| This Model is valid for Automotive grade 3 grade Temperature Range -40C<=Tc<=95C
| Valid for DDR3/DDR3L-1866/2133 operation
| Part Number   VDDQ   Package   Architecture
| SCB13H2G160GF   1.35 +0.1/-0.067   BGA   2G bit x 16
| SCB15H2G160GF   1.5  +0.075/-0.075   BGA   2G bit x 16
[IBIS ver] 5.0
[File name]  ussxh2g16ga3.ibs
[File Rev]  1.0
[Date]   April 23, 2024
[Source] Simulation of a silicon level SPICE model
[Notes]  IBIS Characteristics for I/O Buffer
  IBIS Model Revision History: Rev 1.0:
  2024-04-23 - IBIS model file initial creation
[Disclaimer]  The IBIS models are for modeling purpose only and are subject to change without any notice. UniIC is not
  responsible for any problems the models may cause.
[Copyright] Copyright 2024 UniIC Semiconductors Corp. All rights reserved
|   Component SCB13H2G160GF
[Component] SCB13H2G160GF
[Manufacturer] UniIC Semiconductors Corp.
[Package]
| variable   typ   min   max
R_pkg   0.767   0.689   0.873
L_pkg   2.690nH   2.450nH   3.190nH
C_pkg   0.644pF   0.547pF   0.754pF
[Pin]  signal_name   model_name   R_pin   L_pin   C_pin
A1   VDDQ   Power
A2   DQU5   DQ   0.873   3.190nH   0.754pF
A3   DQU7   DQ   0.808   2.940nH   0.688pF
A7   DQU4   DQ   0.783   2.690nH   0.710pF
A8   VDDQ   Power
A9   VSS   Gnd
B1   VSS   Gnd
B2   VDD   Power
B3   VSS   Gnd
B7   DQSU#   DQ   0.767   2.730nH   0.704pF
B8   DQU6   DQ   0.826   2.890nH   0.738pF
B9   VSS   Gnd
C1   VDDQ   Power
C2   DQU3   DQ   0.800   2.760nH   0.697pF
C3   DQU1   DQ   0.759   2.780nH   0.662pF
C7   DQSU   DQ   0.729   2.680nH   0.650pF
C8   DQU2   DQ   0.739   2.750nH   0.657pF
C9   VDDQ   Power
D1   VSS   Gnd
D2   VDDQ   Power
D3   DMU   DQ   0.730   2.620nH   0.614pF
D7   DQU0   DQ   0.719   2.540nH   0.621pF
D8   VSS   Gnd
D9   VDD   Power
E1   VSS   Gnd
E2   VSS   Gnd
E3   DQL0   DQ   0.777   2.840nH   0.606pF
E7   DML   DQ   0.723   2.480nH   0.608pF
E8   VSS   Gnd
E9   VDDQ   Power
F1   VDDQ   Power
F2   DQL2   DQ   0.738   2.720nH   0.592pF
F3   DQSL   DQ   0.710   2.520nH   0.547pF
F7   DQL1   DQ   0.776   2.590nH   0.556pF
F8   DQL3   DQ   0.793   2.700nH   0.670pF
F9   VSS   Gnd
G1   VSS   Gnd
G2   DQL6   DQ   0.791   2.690nH   0.671pF
G3   DQSL#   DQ   0.689   2.450nH   0.550pF
G7   VDD   Power
G8   VSS   Gnd
G9   VSS   Gnd
H1   VREFDQ   Power
H2   VDDQ   Power
H3   DQL4   DQ   0.740   2.670nH   0.593pF
H7   DQL7   DQ   0.767   2.510nH   0.637pF
H8   DQL5   DQ   0.771   2.560nH   0.629pF
H9   VDDQ   Power
J1   NC1   NC
J2   VSS   Gnd
J3   RAS#   CA   0.738   2.460nH   0.669pF
J7   CK   CLK   0.416   1.450nH   0.409pF
J8   VSS   Gnd
J9   NC2   NC
K1   ODT   RCV_ODT   0.658   2.580nH   0.566pF
K2   VDD   Power
K3   CAS#   CA   0.762   2.490nH   0.692pF
K7   CK#   CLK   0.400   1.490nH   0.364pF
K8   VDD   Power
K9   CKE   CA   0.646   2.440nH   0.567pF
L1   NC3   NC
L2   CS#   CA   0.740   2.760nH   0.578pF
L3   WE#   CA   0.708   2.610nH   0.518pF
L7   A10_AP   CA   0.694   2.670nH   0.504pF
L8   ZQ   Power
L9   NC4   NC
M1   VSS   Gnd
M2   BA0   CA   0.762   3.000nH   0.609pF
M3   BA2   CA   0.725   2.790nH   0.545pF
M7   NC5   NC
M8   VREFCA   Power
M9   VSS   Gnd
N1   VDD   Power
N2   A3   CA   0.697   2.800nH   0.595pF
N3   A0   CA   0.654   2.720nH   0.550pF
N7   A12_BC   CA   0.691   2.550nH   0.585pF
N8   BA1   CA   0.734   3.070nH   0.562pF
N9   VDD   Power
P1   VSS   Gnd
P2   A5   CA   0.723   2.950nH   0.631pF
P3   A2   CA   0.725   2.990nH   0.598pF
P7   A1   CA   0.641   2.670nH   0.572pF
P8   A4   CA   0.721   2.780nH   0.646pF
P9   VSS   Gnd
R1   VDD   Power
R2   A7   CA   0.801   3.060nH   0.699pF
R3   A9   CA   0.712   2.920nH   0.627pF
R7   A11   CA   0.677   2.830nH   0.602pF
R8   A6   CA   0.793   3.120nH   0.708pF
R9   VDD   Power
T1   VSS   Gnd
T2   RESET#   RST_N
T3   A13   CA   0.807   2.990nH   0.695pF
T7   NC6   NC
T8   A8   CA   0.867   3.280nH   0.754pF
T9   VSS   Gnd
|IN   dq_in   dummy
|EN   dq_en   dummy
[Diff pin]  inv_pin  vdiff   tdelay_typ   tdelay_min   tdelay_max
C7   B7   0.270V   NA   NA   NA
F3   G3   0.270V   NA   NA   NA
J7   K7   0.270V   NA   NA   NA
|   Component SCB15H2G160GF
[Component] SCB15H2G160GF
[Manufacturer] UniIC Semiconductors Corp.
[Package]
| variable   typ   min   max
R_pkg   0.767   0.689   0.873
L_pkg   2.690nH   2.450nH   3.190nH
C_pkg   0.644pF   0.547pF   0.754pF
[Pin]  signal_name   model_name   R_pin   L_pin   C_pin
A1   VDDQ   Power
A2   DQU5   DQ   0.873   3.190nH   0.754pF
A3   DQU7   DQ   0.808   2.940nH   0.688pF
A7   DQU4   DQ   0.783   2.690nH   0.710pF
A8   VDDQ   Power
A9   VSS   Gnd
B1   VSS   Gnd
B2   VDD   Power
B3   VSS   Gnd
B7   DQSU#   DQ   0.767   2.730nH   0.704pF
B8   DQU6   DQ   0.826   2.890nH   0.738pF
B9   VSS   Gnd
C1   VDDQ   Power
C2   DQU3   DQ   0.800   2.760nH   0.697pF
C3   DQU1   DQ   0.759   2.780nH   0.662pF
C7   DQSU   DQ   0.729   2.680nH   0.650pF
C8   DQU2   DQ   0.739   2.750nH   0.657pF
C9   VDDQ   Power
D1   VSS   Gnd
D2   VDDQ   Power
D3   DMU   DQ   0.730   2.620nH   0.614pF
D7   DQU0   DQ   0.719   2.540nH   0.621pF
D8   VSS   Gnd
D9   VDD   Power
E1   VSS   Gnd
E2   VSS   Gnd
E3   DQL0   DQ   0.777   2.840nH   0.606pF
E7   DML   DQ   0.723   2.480nH   0.608pF
E8   VSS   Gnd
E9   VDDQ   Power
F1   VDDQ   Power
F2   DQL2   DQ   0.738   2.720nH   0.592pF
F3   DQSL   DQ   0.710   2.520nH   0.547pF
F7   DQL1   DQ   0.776   2.590nH   0.556pF
F8   DQL3   DQ   0.793   2.700nH   0.670pF
F9   VSS   Gnd
G1   VSS   Gnd
G2   DQL6   DQ   0.791   2.690nH   0.671pF
G3   DQSL#   DQ   0.689   2.450nH   0.550pF
G7   VDD   Power
G8   VSS   Gnd
G9   VSS   Gnd
H1   VREFDQ   Power
H2   VDDQ   Power
H3   DQL4   DQ   0.740   2.670nH   0.593pF
H7   DQL7   DQ   0.767   2.510nH   0.637pF
H8   DQL5   DQ   0.771   2.560nH   0.629pF
H9   VDDQ   Power
J1   NC1   NC
J2   VSS   Gnd
J3   RAS#   CA   0.738   2.460nH   0.669pF
J7   CK   CLK   0.416   1.450nH   0.409pF
J8   VSS   Gnd
J9   NC2   NC
K1   ODT   RCV_ODT   0.658   2.580nH   0.566pF
K2   VDD   Power
K3   CAS#   CA   0.762   2.490nH   0.692pF
K7   CK#   CLK   0.400   1.490nH   0.364pF
K8   VDD   Power
K9   CKE   CA   0.646   2.440nH   0.567pF
L1   NC3   NC
L2   CS#   CA   0.740   2.760nH   0.578pF
L3   WE#   CA   0.708   2.610nH   0.518pF
L7   A10_AP   CA   0.694   2.670nH   0.504pF
L8   ZQ   Power
L9   NC4   NC
M1   VSS   Gnd
M2   BA0   CA   0.762   3.000nH   0.609pF
M3   BA2   CA   0.725   2.790nH   0.545pF
M7   NC5   NC
M8   VREFCA   Power
M9   VSS   Gnd
N1   VDD   Power
N2   A3   CA   0.697   2.800nH   0.595pF
N3   A0   CA   0.654   2.720nH   0.550pF
N7   A12_BC   CA   0.691   2.550nH   0.585pF
N8   BA1   CA   0.734   3.070nH   0.562pF
N9   VDD   Power
P1   VSS   Gnd
P2   A5   CA   0.723   2.950nH   0.631pF
P3   A2   CA   0.725   2.990nH   0.598pF
P7   A1   CA   0.641   2.670nH   0.572pF
P8   A4   CA   0.721   2.780nH   0.646pF
P9   VSS   Gnd
R1   VDD   Power
R2   A7   CA   0.801   3.060nH   0.699pF
R3   A9   CA   0.712   2.920nH   0.627pF
R7   A11   CA   0.677   2.830nH   0.602pF
R8   A6   CA   0.793   3.120nH   0.708pF
R9   VDD   Power
T1   VSS   Gnd
T2   RESET#   RST_N
T3   A13   CA   0.807   2.990nH   0.695pF
T7   NC6   NC
T8   A8   CA   0.867   3.280nH   0.754pF
T9   VSS   Gnd
[Diff pin]  inv_pin  vdiff   tdelay_typ   tdelay_min   tdelay_max
C7   B7   0.270V   NA   NA   NA
F3   G3   0.270V   NA   NA   NA
J7   K7   0.270V   NA   NA   NA
[Model Selector] DQ
DQ_RON60_DDR3  DQ/ DQS RON=60ohms, for DDR3
DQ_RON60_DDR3L  DQ/ DQS RON=60ohms, for DDR3L
DQ_RON48_DDR3  DQ/ DQS RON=48ohms, for DDR3
DQ_RON48_DDR3L  DQ/ DQS RON=48ohms, for DDR3L
DQ_RON40_DDR3  DQ/ DQS RON=40ohms, for DDR3
DQ_RON40_DDR3L  DQ/ DQS RON=40ohms, for DDR3L
DQ_RON34_DDR3  DQ/ DQS RON=34ohms, for DDR3
DQ_RON34_DDR3L  DQ/ DQS RON=34ohms, for DDR3L
DQ_RCV_ODTOFF_DDR3  DQ/DM RCV ODTOFF, for DDR3
DQ_RCV_ODTOFF_DDR3L  DQ/DM RCV ODTOFF, for DDR3L
DQ_RCV_ODT120_DDR3  DQ/DM RCV ODT120, for DDR3
DQ_RCV_ODT120_DDR3L  DQ/DM RCV ODT120, for DDR3L
DQ_RCV_ODT60_DDR3  DQ/DM RCV ODT60, for DDR3
DQ_RCV_ODT60_DDR3L  DQ/DM RCV ODT60, for DDR3L
DQ_RCV_ODT40_DDR3  DQ/DM RCV ODT40, for DDR3
DQ_RCV_ODT40_DDR3L  DQ/DM RCV ODT40, for DDR3L
DQ_RCV_ODT30_DDR3  DQ/DM RCV ODT30, for DDR3
DQ_RCV_ODT30_DDR3L  DQ/DM RCV ODT30, for DDR3L
DQ_RCV_ODT20_DDR3  DQ/DM RCV ODT20, for DDR3
DQ_RCV_ODT20_DDR3L  DQ/DM RCV ODT20, for DDR3L
[Model Selector] CLK
RCV_CLK_DDR3  RCV_CKC/CKT for DDR3
RCV_CLK_DDR3L  RCV_CKC/CKT for DDR3L
[Model Selector] CA
RCV_CA_DDR3  RCV_CA/BA/CS_N/CKE/CAS_N/RAS_N/WE_N for DDR3
RCV_CA_DDR3L  RCV_CA/BA/CS_N/CKE/CAS_N/RAS_N/WE_N for DDR3L
[Model Selector] RCV_ODT
RCV_ODT_DDR3  RCV_ODT for DDR3
RCV_ODT_DDR3L  RCV_ODT for DDR3L
[Model Selector] RST_N
RCV_RST_N_DDR3  RCV RST_N for DDR3
RCV_RST_N_DDR3L  RCV RST_N for DDR3L
| Models and submodels in the file (28): DQ_RON60_DDR3 (I/O), DQ_RON60_DDR3L (I/O), DQ_RON48_DDR3 (I/O), DQ_RON48_DDR3L (I/O), DQ_RON40_DDR3 (I/O), DQ_RON40_DDR3L (I/O), DQ_RON34_DDR3 (I/O), DQ_RON34_DDR3L (I/O), DQ_RCV_ODTOFF_DDR3 (Input), DQ_RCV_ODTOFF_DDR3L (Input), DQ_RCV_ODT120_DDR3 (Input), DQ_RCV_ODT120_DDR3L (Input), DQ_RCV_ODT60_DDR3 (Input), DQ_RCV_ODT60_DDR3L (Input), DQ_RCV_ODT40_DDR3 (Input), DQ_RCV_ODT40_DDR3L (Input), DQ_RCV_ODT30_DDR3 (Input), DQ_RCV_ODT30_DDR3L (Input), DQ_RCV_ODT20_DDR3 (Input), DQ_RCV_ODT20_DDR3L (Input), RCV_CLK_DDR3 (Input), RCV_CLK_DDR3L (Input), RCV_CA_DDR3 (Input), RCV_CA_DDR3L (Input), RCV_ODT_DDR3 (Input), RCV_ODT_DDR3L (Input), RCV_RST_N_DDR3 (Input), RCV_RST_N_DDR3L (Input)
